(* Logix 5000 AddOnInstructionDefinition export Banner_Q90RKU_Param_v4; software revision 33.00; part 2 of 2 *)
(* tags used below, declared in another part *)
   Q90RKU : Banner_Q90RKU_v4;
   Port_Data : Banner_IOL_Port_v4;
   Port : DINT;
   Local_Control : DINT;
   Command_Being_Processed : BOOL;
   Update_Archive : BOOL;
   Index_Write_Inprocess : DINT;
   Index_Write_Control : DINT;
   Inprocess_Index : DINT;
(* Banner_Q90RKU_Param_v4, continued *)

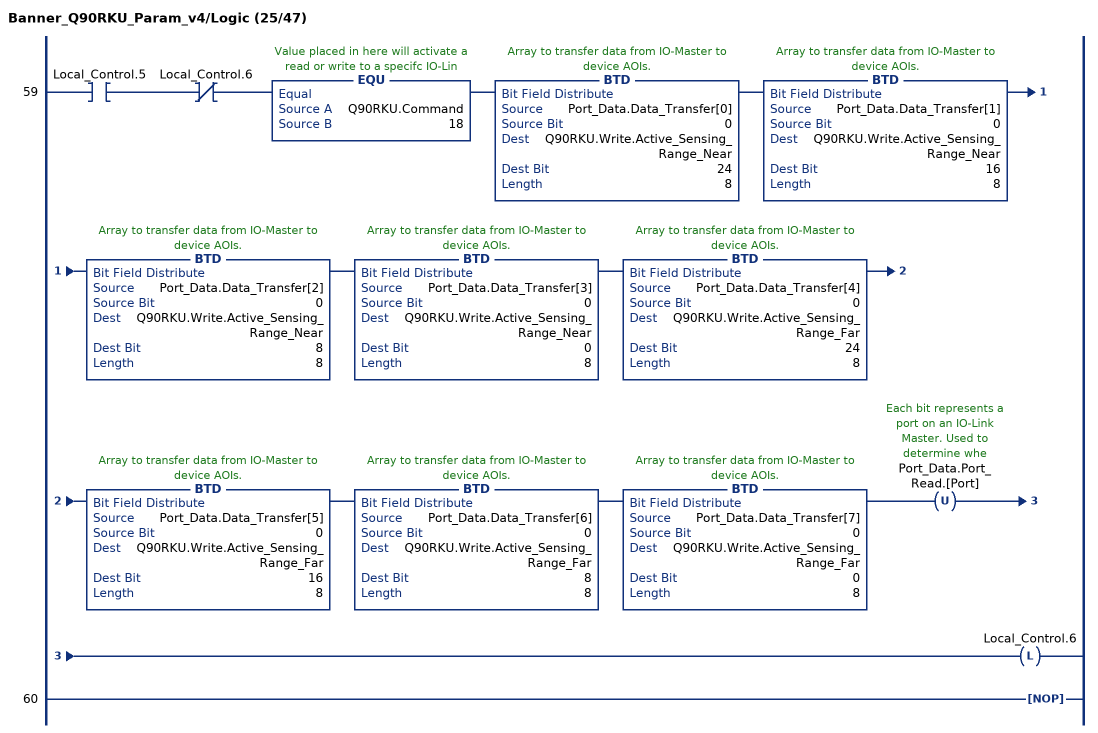
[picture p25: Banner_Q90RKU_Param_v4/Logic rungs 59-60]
   59: XIC(Local_Control.5)XIO(Local_Control.6)EQU(Q90RKU.Command,18)BTD(Port_Data.Data_Transfer[0],0,Q90RKU.Write.Active_Sensing_Range_Near,24,8)BTD(Port_Data.Data_Transfer[1],0,Q90RKU.Write.Active_Sensing_Range_Near,16,8)BTD(Port_Data.Data_Transfer[2],0,Q90RKU.Write.Active_Sensing_Range_Near,8,8)BTD(Port_Data.Data_Transfer[3],0,Q90RKU.Write.Active_Sensing_Range_Near,0,8)BTD(Port_Data.Data_Transfer[4],0,Q90RKU.Write.Active_Sensing_Range_Far,24,8)BTD(Port_Data.Data_Transfer[5],0,Q90RKU.Write.Active_Sensing_Range_Far,16,8)BTD(Port_Data.Data_Transfer[6],0,Q90RKU.Write.Active_Sensing_Range_Far,8,8)BTD(Port_Data.Data_Transfer[7],0,Q90RKU.Write.Active_Sensing_Range_Far,0,8)OTU(Port_Data.Port_Read.[Port])OTL(Local_Control.6);
   60: NOP();
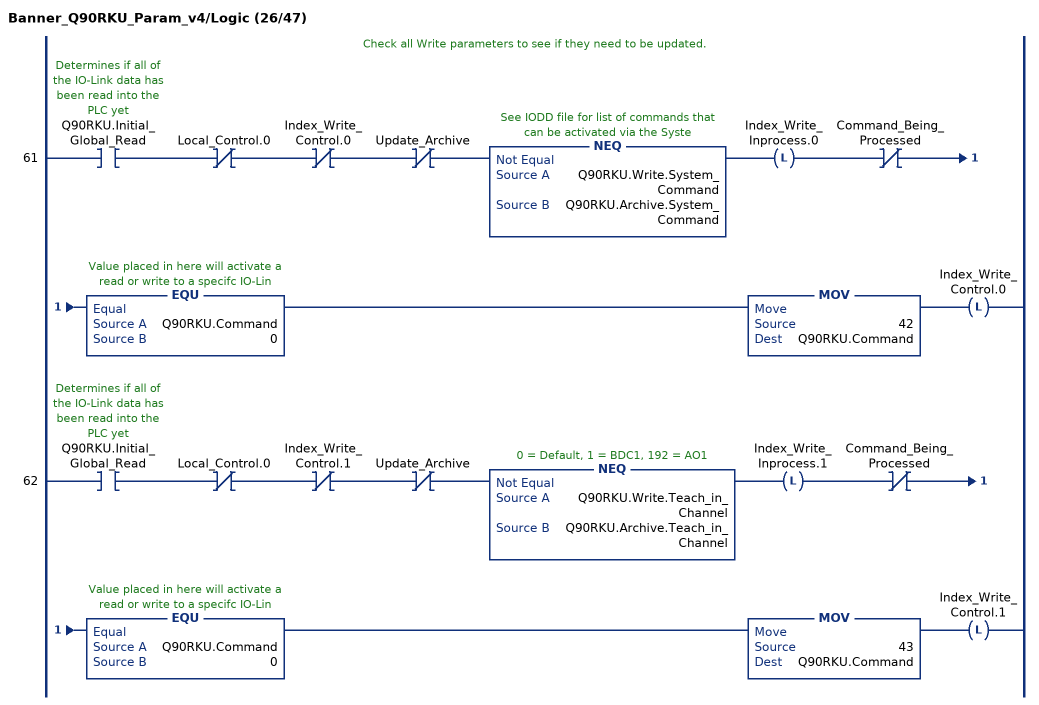
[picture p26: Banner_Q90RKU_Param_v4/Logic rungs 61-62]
   // Check all Write parameters to see if they need to be updated.
   61: XIC(Q90RKU.Initial_Global_Read)XIO(Local_Control.0)XIO(Index_Write_Control.0)XIO(Update_Archive)NEQ(Q90RKU.Write.System_Command,Q90RKU.Archive.System_Command)OTL(Index_Write_Inprocess.0)XIO(Command_Being_Processed)EQU(Q90RKU.Command,0)MOV(42,Q90RKU.Command)OTL(Index_Write_Control.0);
   62: XIC(Q90RKU.Initial_Global_Read)XIO(Local_Control.0)XIO(Index_Write_Control.1)XIO(Update_Archive)NEQ(Q90RKU.Write.Teach_in_Channel,Q90RKU.Archive.Teach_in_Channel)OTL(Index_Write_Inprocess.1)XIO(Command_Being_Processed)EQU(Q90RKU.Command,0)MOV(43,Q90RKU.Command)OTL(Index_Write_Control.1);
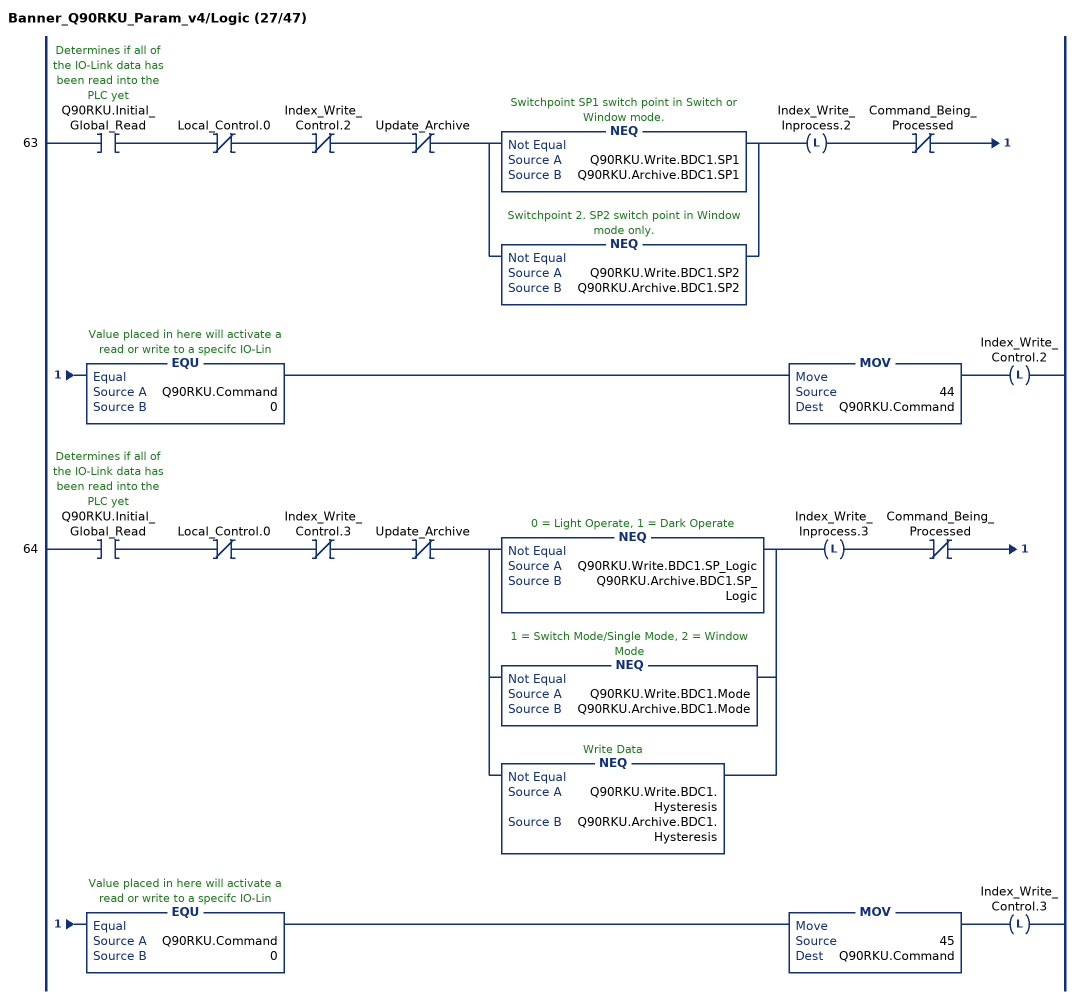
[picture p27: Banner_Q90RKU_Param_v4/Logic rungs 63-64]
   63: XIC(Q90RKU.Initial_Global_Read)XIO(Local_Control.0)XIO(Index_Write_Control.2)XIO(Update_Archive)[NEQ(Q90RKU.Write.BDC1.SP1,Q90RKU.Archive.BDC1.SP1) ,NEQ(Q90RKU.Write.BDC1.SP2,Q90RKU.Archive.BDC1.SP2) ]OTL(Index_Write_Inprocess.2)XIO(Command_Being_Processed)EQU(Q90RKU.Command,0)MOV(44,Q90RKU.Command)OTL(Index_Write_Control.2);
   64: XIC(Q90RKU.Initial_Global_Read)XIO(Local_Control.0)XIO(Index_Write_Control.3)XIO(Update_Archive)[NEQ(Q90RKU.Write.BDC1.SP_Logic,Q90RKU.Archive.BDC1.SP_Logic) ,NEQ(Q90RKU.Write.BDC1.Mode,Q90RKU.Archive.BDC1.Mode) ,NEQ(Q90RKU.Write.BDC1.Hysteresis,Q90RKU.Archive.BDC1.Hysteresis) ]OTL(Index_Write_Inprocess.3)XIO(Command_Being_Processed)EQU(Q90RKU.Command,0)MOV(45,Q90RKU.Command)OTL(Index_Write_Control.3);
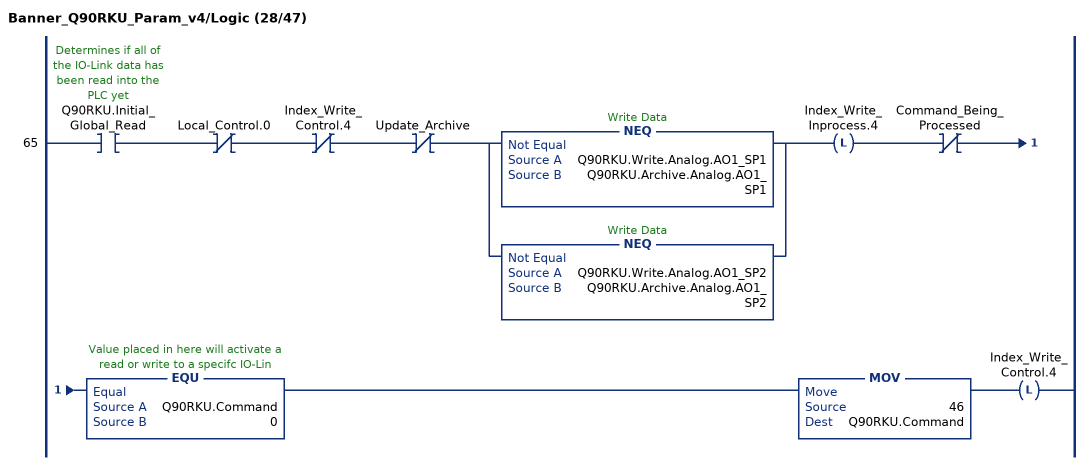
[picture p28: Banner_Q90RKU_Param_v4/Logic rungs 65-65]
   65: XIC(Q90RKU.Initial_Global_Read)XIO(Local_Control.0)XIO(Index_Write_Control.4)XIO(Update_Archive)[NEQ(Q90RKU.Write.Analog.AO1_SP1,Q90RKU.Archive.Analog.AO1_SP1) ,NEQ(Q90RKU.Write.Analog.AO1_SP2,Q90RKU.Archive.Analog.AO1_SP2) ]OTL(Index_Write_Inprocess.4)XIO(Command_Being_Processed)EQU(Q90RKU.Command,0)MOV(46,Q90RKU.Command)OTL(Index_Write_Control.4);
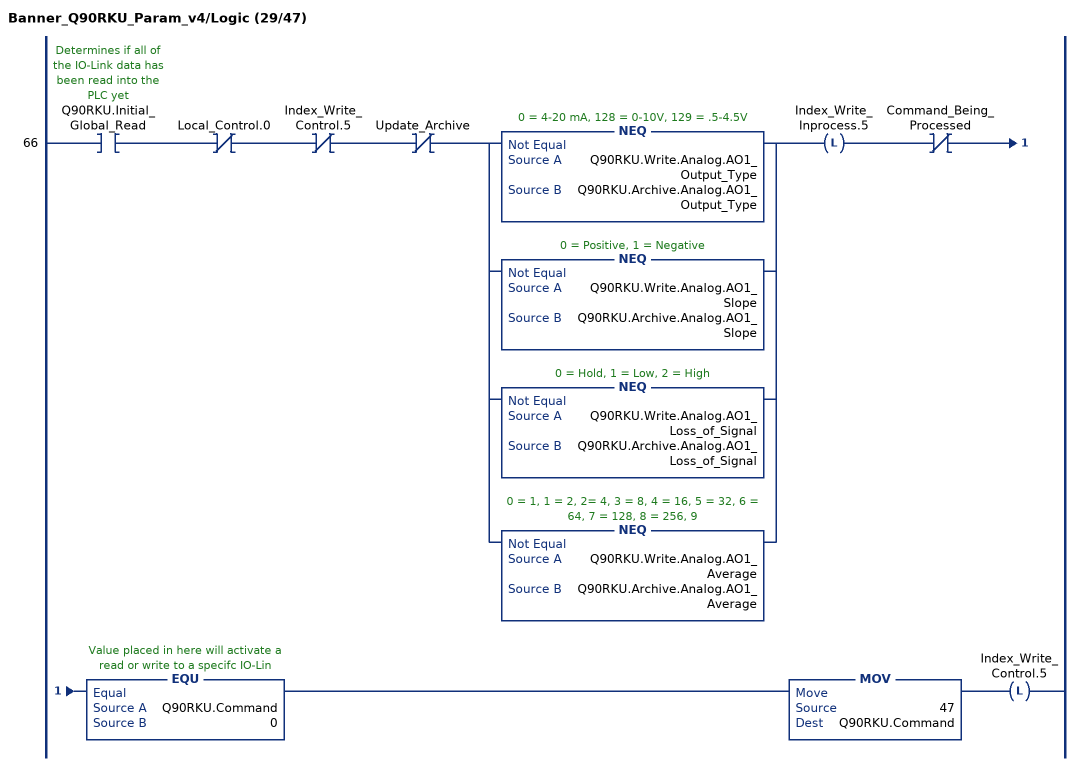
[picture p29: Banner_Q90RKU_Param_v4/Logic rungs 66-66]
   66: XIC(Q90RKU.Initial_Global_Read)XIO(Local_Control.0)XIO(Index_Write_Control.5)XIO(Update_Archive)[NEQ(Q90RKU.Write.Analog.AO1_Output_Type,Q90RKU.Archive.Analog.AO1_Output_Type) ,NEQ(Q90RKU.Write.Analog.AO1_Slope,Q90RKU.Archive.Analog.AO1_Slope) ,NEQ(Q90RKU.Write.Analog.AO1_Loss_of_Signal,Q90RKU.Archive.Analog.AO1_Loss_of_Signal) ,NEQ(Q90RKU.Write.Analog.AO1_Average,Q90RKU.Archive.Analog.AO1_Average) ]OTL(Index_Write_Inprocess.5)XIO(Command_Being_Processed)EQU(Q90RKU.Command,0)MOV(47,Q90RKU.Command)OTL(Index_Write_Control.5);
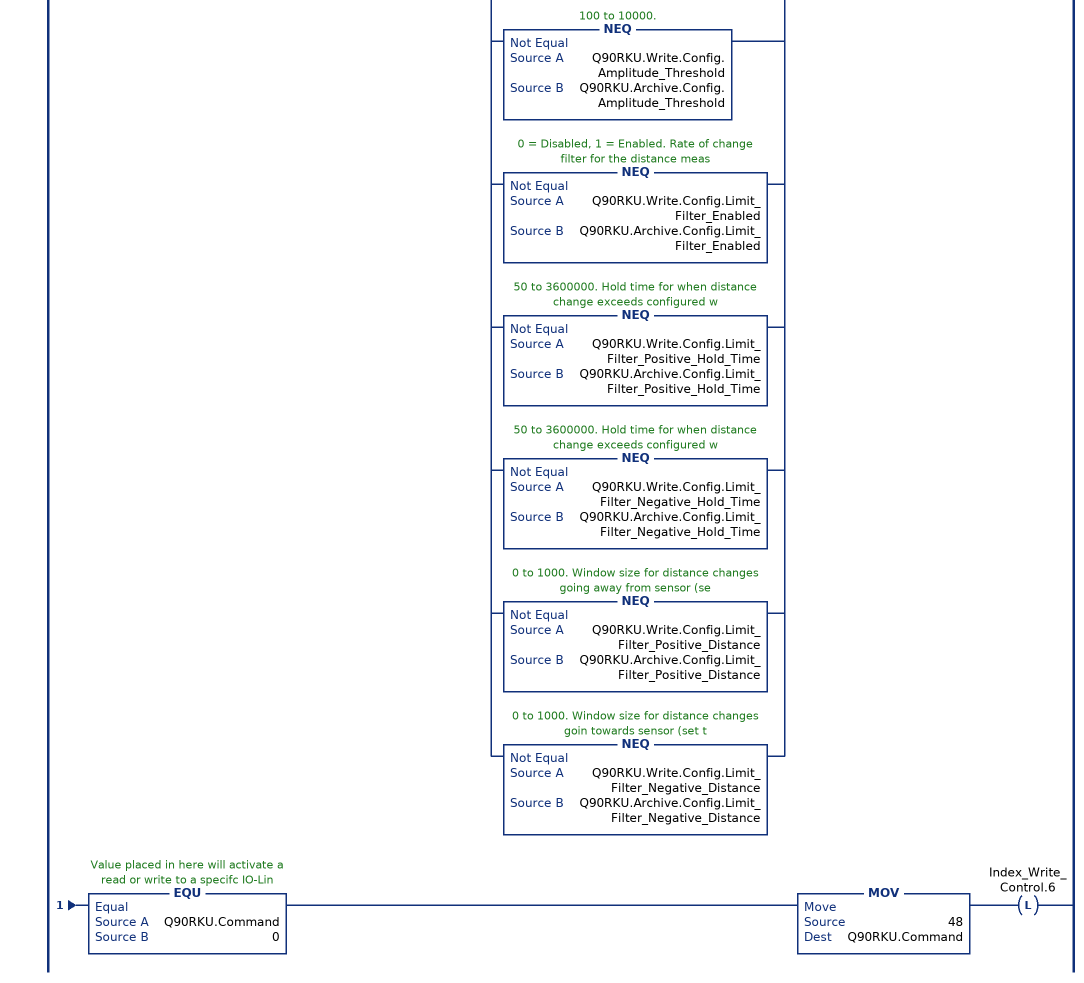
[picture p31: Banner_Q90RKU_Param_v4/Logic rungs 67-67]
   67: XIC(Q90RKU.Initial_Global_Read)XIO(Local_Control.0)XIO(Index_Write_Control.6)XIO(Update_Archive)[NEQ(Q90RKU.Write.Config.Response_Speed,Q90RKU.Archive.Config.Response_Speed) ,NEQ(Q90RKU.Write.Config.Peak_Select_Mode,Q90RKU.Archive.Config.Peak_Select_Mode) ,NEQ(Q90RKU.Write.Config.Output_Polarity,Q90RKU.Archive.Config.Output_Polarity) ,NEQ(Q90RKU.Write.Config.Process_Data_Filter_Time,Q90RKU.Archive.Config.Process_Data_Filter_Time) ,NEQ(Q90RKU.Write.Config.Process_Data_Layout,Q90RKU.Archive.Config.Process_Data_Layout) ,NEQ(Q90RKU.Write.Config.Remote_Input_Mode,Q90RKU.Archive.Config.Remote_Input_Mode) ,NEQ(Q90RKU.Write.Config.LEDs_Disabled,Q90RKU.Archive.Config.LEDs_Disabled) ,NEQ(Q90RKU.Write.Config.Amplitude_Threshold,Q90RKU.Archive.Config.Amplitude_Threshold) ,NEQ(Q90RKU.Write.Config.Limit_Filter_Enabled,Q90RKU.Archive.Config.Limit_Filter_Enabled) ,NEQ(Q90RKU.Write.Config.Limit_Filter_Positive_Hold_Time,Q90RKU.Archive.Config.Limit_Filter_Positive_Hold_Time) ,NEQ(Q90RKU.Write.Config.Limit_Filter_Negative_Hold_Time,Q90RKU.Archive.Config.Limit_Filter_Negative_Hold_Time) ,NEQ(Q90RKU.Write.Config.Limit_Filter_Positive_Distance,Q90RKU.Archive.Config.Limit_Filter_Positive_Distance) ,NEQ(Q90RKU.Write.Config.Limit_Filter_Negative_Distance,Q90RKU.Archive.Config.Limit_Filter_Negative_Distance) ]OTL(Index_Write_Inprocess.6)XIO(Command_Being_Processed)EQU(Q90RKU.Command,0)MOV(48,Q90RKU.Command)OTL(Index_Write_Control.6);
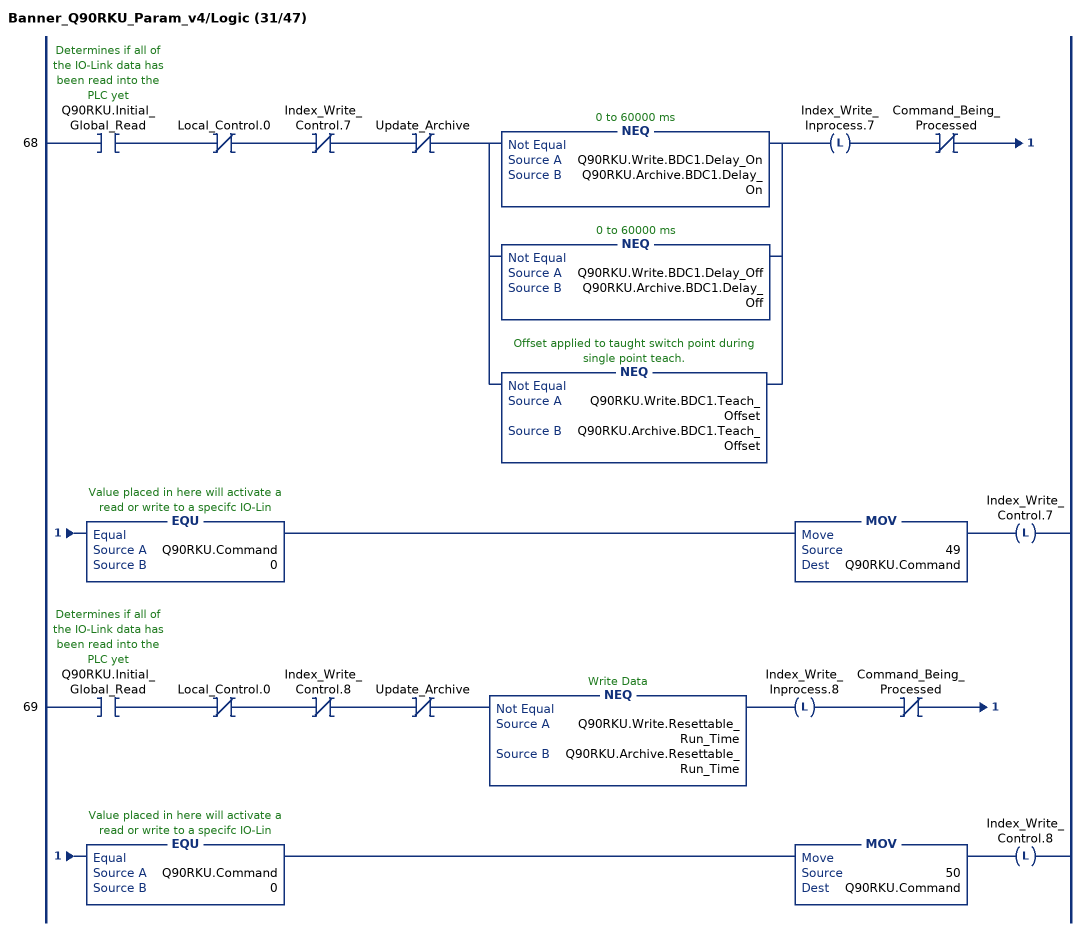
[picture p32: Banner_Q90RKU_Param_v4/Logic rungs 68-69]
   68: XIC(Q90RKU.Initial_Global_Read)XIO(Local_Control.0)XIO(Index_Write_Control.7)XIO(Update_Archive)[NEQ(Q90RKU.Write.BDC1.Delay_On,Q90RKU.Archive.BDC1.Delay_On) ,NEQ(Q90RKU.Write.BDC1.Delay_Off,Q90RKU.Archive.BDC1.Delay_Off) ,NEQ(Q90RKU.Write.BDC1.Teach_Offset,Q90RKU.Archive.BDC1.Teach_Offset) ]OTL(Index_Write_Inprocess.7)XIO(Command_Being_Processed)EQU(Q90RKU.Command,0)MOV(49,Q90RKU.Command)OTL(Index_Write_Control.7);
   69: XIC(Q90RKU.Initial_Global_Read)XIO(Local_Control.0)XIO(Index_Write_Control.8)XIO(Update_Archive)NEQ(Q90RKU.Write.Resettable_Run_Time,Q90RKU.Archive.Resettable_Run_Time)OTL(Index_Write_Inprocess.8)XIO(Command_Being_Processed)EQU(Q90RKU.Command,0)MOV(50,Q90RKU.Command)OTL(Index_Write_Control.8);
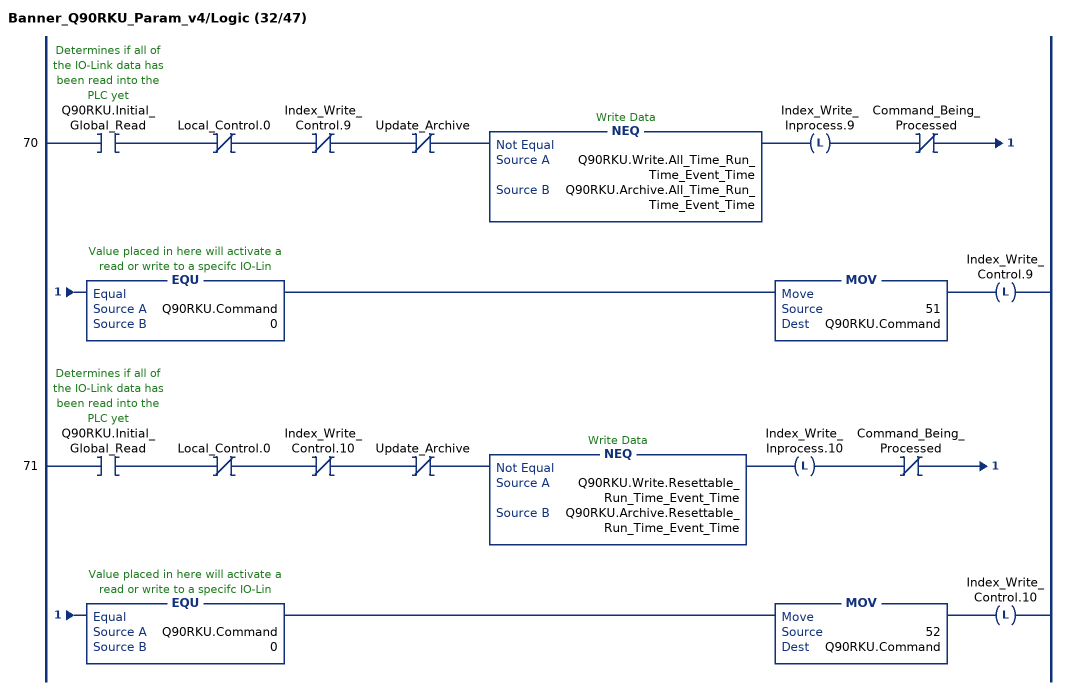
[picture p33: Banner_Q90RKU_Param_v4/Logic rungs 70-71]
   70: XIC(Q90RKU.Initial_Global_Read)XIO(Local_Control.0)XIO(Index_Write_Control.9)XIO(Update_Archive)NEQ(Q90RKU.Write.All_Time_Run_Time_Event_Time,Q90RKU.Archive.All_Time_Run_Time_Event_Time)OTL(Index_Write_Inprocess.9)XIO(Command_Being_Processed)EQU(Q90RKU.Command,0)MOV(51,Q90RKU.Command)OTL(Index_Write_Control.9);
   71: XIC(Q90RKU.Initial_Global_Read)XIO(Local_Control.0)XIO(Index_Write_Control.10)XIO(Update_Archive)NEQ(Q90RKU.Write.Resettable_Run_Time_Event_Time,Q90RKU.Archive.Resettable_Run_Time_Event_Time)OTL(Index_Write_Inprocess.10)XIO(Command_Being_Processed)EQU(Q90RKU.Command,0)MOV(52,Q90RKU.Command)OTL(Index_Write_Control.10);
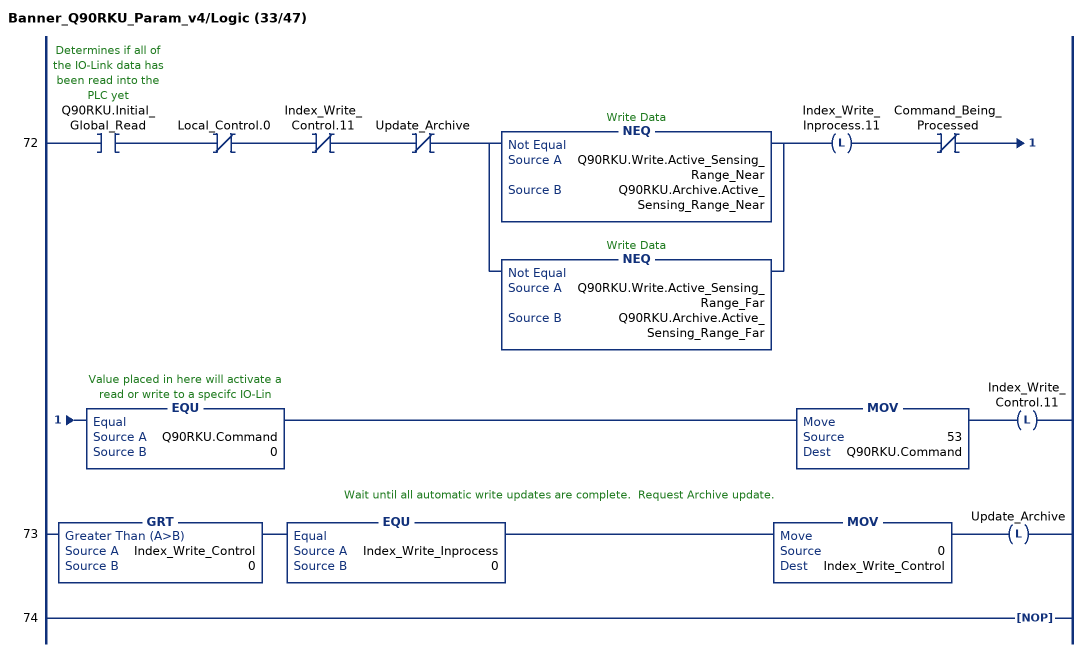
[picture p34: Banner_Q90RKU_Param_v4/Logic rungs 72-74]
   72: XIC(Q90RKU.Initial_Global_Read)XIO(Local_Control.0)XIO(Index_Write_Control.11)XIO(Update_Archive)[NEQ(Q90RKU.Write.Active_Sensing_Range_Near,Q90RKU.Archive.Active_Sensing_Range_Near) ,NEQ(Q90RKU.Write.Active_Sensing_Range_Far,Q90RKU.Archive.Active_Sensing_Range_Far) ]OTL(Index_Write_Inprocess.11)XIO(Command_Being_Processed)EQU(Q90RKU.Command,0)MOV(53,Q90RKU.Command)OTL(Index_Write_Control.11);
   // Wait until all automatic write updates are complete.  Request Archive update.
   73: GRT(Index_Write_Control,0)EQU(Index_Write_Inprocess,0)MOV(0,Index_Write_Control)OTL(Update_Archive);
   74: NOP();
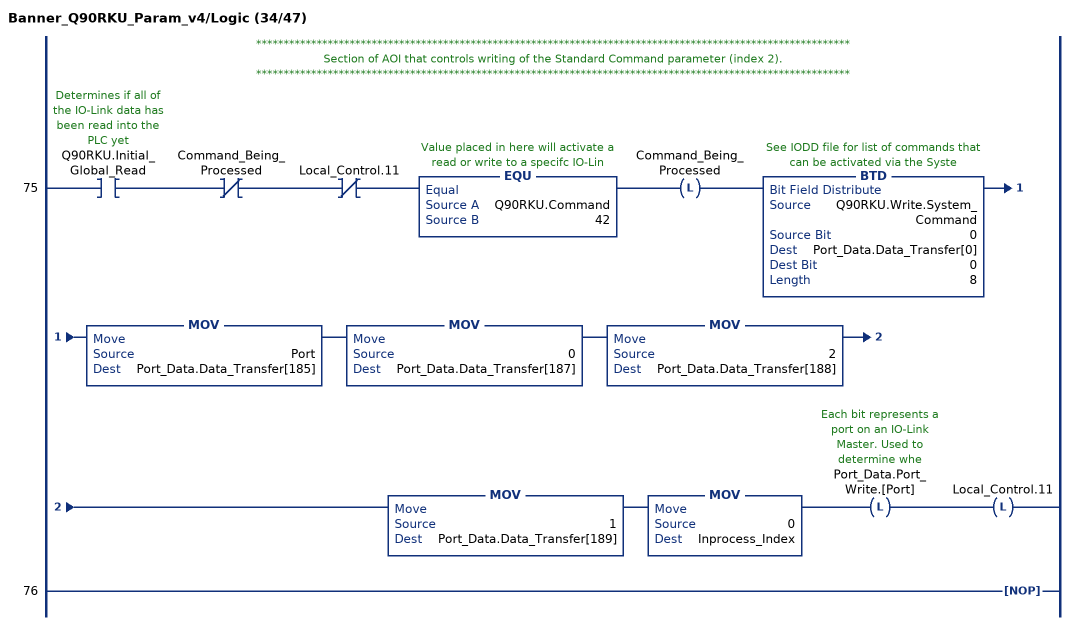
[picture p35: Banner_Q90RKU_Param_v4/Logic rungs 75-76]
   // ************************************************************************************************************
   // Section of AOI that controls writing of the Standard Command parameter (index 2).
   // ************************************************************************************************************
   75: XIC(Q90RKU.Initial_Global_Read)XIO(Command_Being_Processed)XIO(Local_Control.11)EQU(Q90RKU.Command,42)OTL(Command_Being_Processed)BTD(Q90RKU.Write.System_Command,0,Port_Data.Data_Transfer[0],0,8)MOV(Port,Port_Data.Data_Transfer[185])MOV(0,Port_Data.Data_Transfer[187])MOV(2,Port_Data.Data_Transfer[188])MOV(1,Port_Data.Data_Transfer[189])MOV(0,Inprocess_Index)OTL(Port_Data.Port_Write.[Port])OTL(Local_Control.11);
   76: NOP();
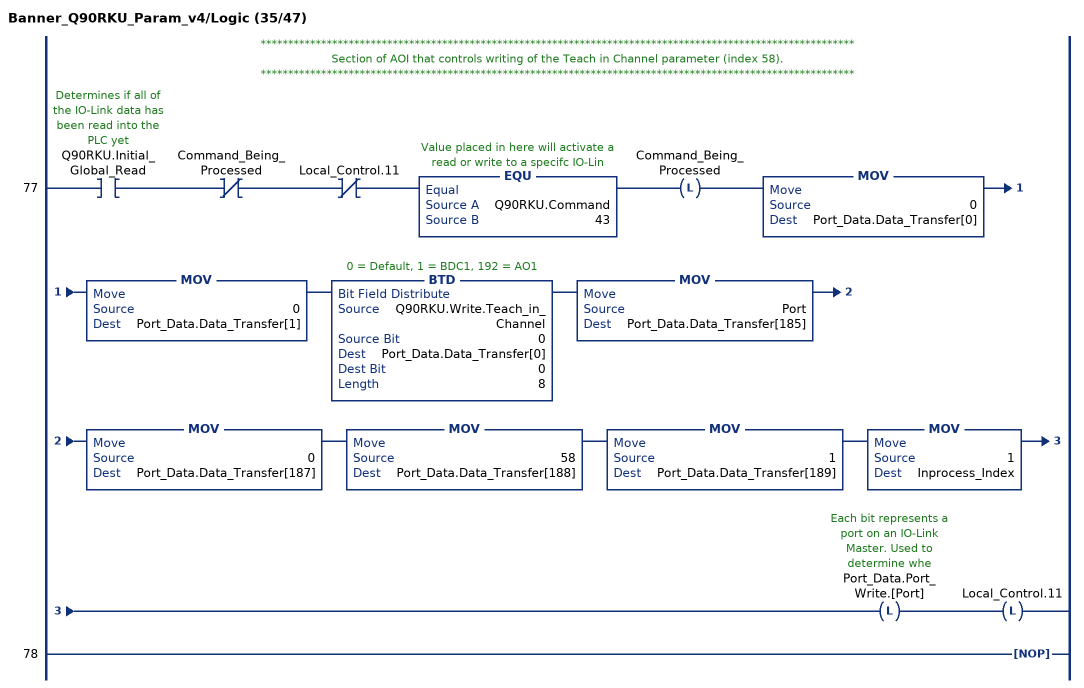
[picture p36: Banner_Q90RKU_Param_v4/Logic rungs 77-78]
   // ************************************************************************************************************
   // Section of AOI that controls writing of the Teach in Channel parameter (index 58).
   // ************************************************************************************************************
   77: XIC(Q90RKU.Initial_Global_Read)XIO(Command_Being_Processed)XIO(Local_Control.11)EQU(Q90RKU.Command,43)OTL(Command_Being_Processed)MOV(0,Port_Data.Data_Transfer[0])MOV(0,Port_Data.Data_Transfer[1])BTD(Q90RKU.Write.Teach_in_Channel,0,Port_Data.Data_Transfer[0],0,8)MOV(Port,Port_Data.Data_Transfer[185])MOV(0,Port_Data.Data_Transfer[187])MOV(58,Port_Data.Data_Transfer[188])MOV(1,Port_Data.Data_Transfer[189])MOV(1,Inprocess_Index)OTL(Port_Data.Port_Write.[Port])OTL(Local_Control.11);
   78: NOP();
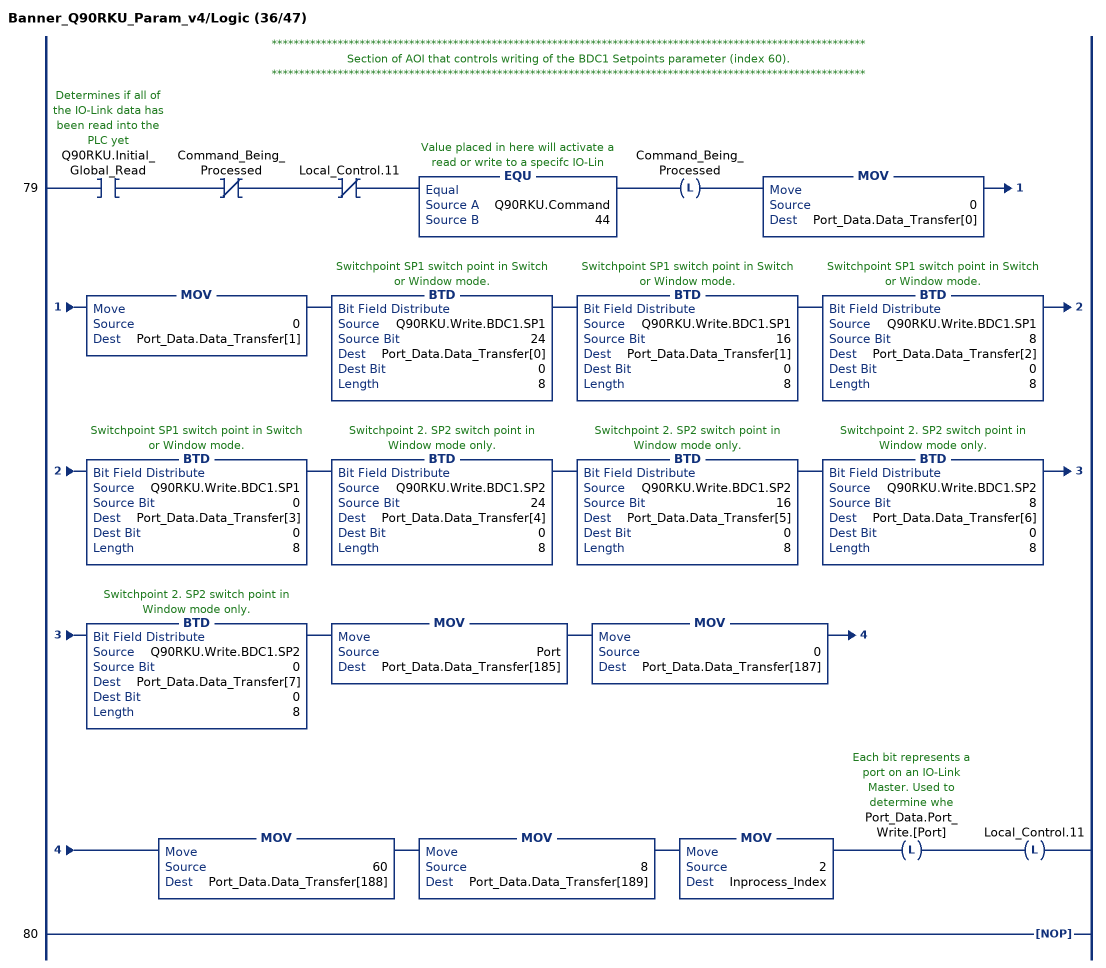
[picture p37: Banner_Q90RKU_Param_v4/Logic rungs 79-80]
   // ************************************************************************************************************
   // Section of AOI that controls writing of the BDC1 Setpoints parameter (index 60).
   // ************************************************************************************************************
   79: XIC(Q90RKU.Initial_Global_Read)XIO(Command_Being_Processed)XIO(Local_Control.11)EQU(Q90RKU.Command,44)OTL(Command_Being_Processed)MOV(0,Port_Data.Data_Transfer[0])MOV(0,Port_Data.Data_Transfer[1])BTD(Q90RKU.Write.BDC1.SP1,24,Port_Data.Data_Transfer[0],0,8)BTD(Q90RKU.Write.BDC1.SP1,16,Port_Data.Data_Transfer[1],0,8)BTD(Q90RKU.Write.BDC1.SP1,8,Port_Data.Data_Transfer[2],0,8)BTD(Q90RKU.Write.BDC1.SP1,0,Port_Data.Data_Transfer[3],0,8)BTD(Q90RKU.Write.BDC1.SP2,24,Port_Data.Data_Transfer[4],0,8)BTD(Q90RKU.Write.BDC1.SP2,16,Port_Data.Data_Transfer[5],0,8)BTD(Q90RKU.Write.BDC1.SP2,8,Port_Data.Data_Transfer[6],0,8)BTD(Q90RKU.Write.BDC1.SP2,0,Port_Data.Data_Transfer[7],0,8)MOV(Port,Port_Data.Data_Transfer[185])MOV(0,Port_Data.Data_Transfer[187])MOV(60,Port_Data.Data_Transfer[188])MOV(8,Port_Data.Data_Transfer[189])MOV(2,Inprocess_Index)OTL(Port_Data.Port_Write.[Port])OTL(Local_Control.11);
   80: NOP();
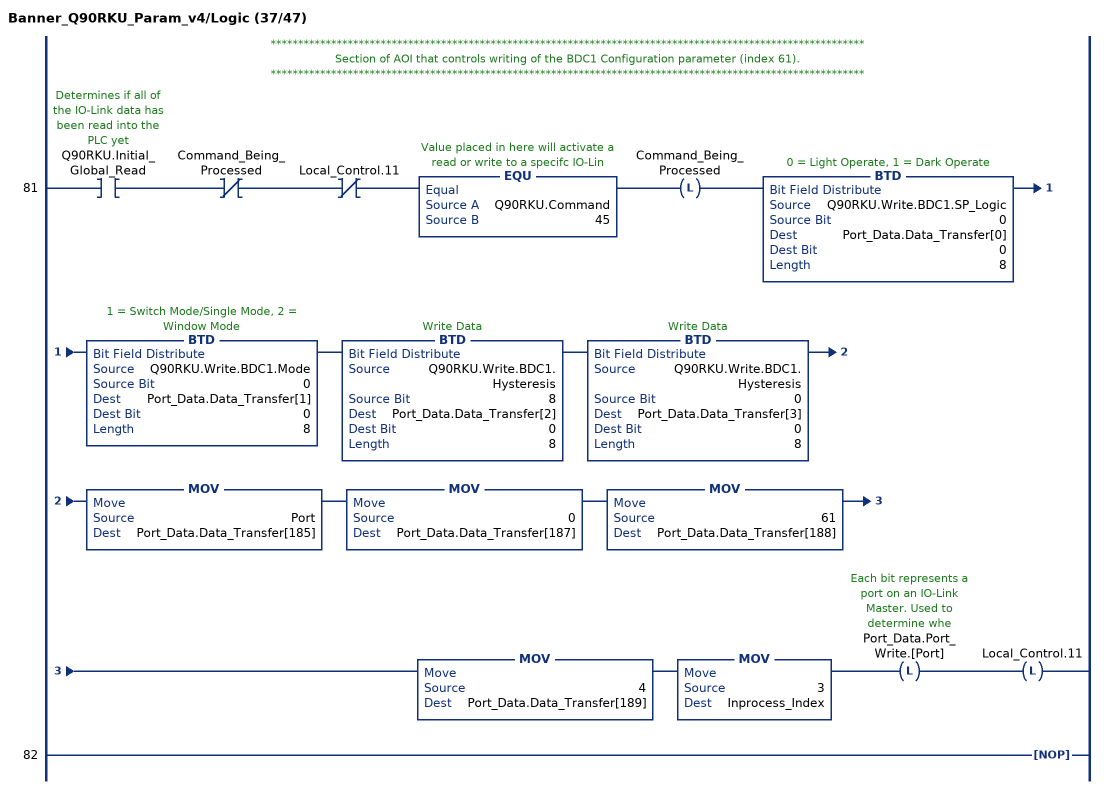
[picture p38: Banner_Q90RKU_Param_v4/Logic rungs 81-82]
   // ************************************************************************************************************
   // Section of AOI that controls writing of the BDC1 Configuration parameter (index 61).
   // ************************************************************************************************************
   81: XIC(Q90RKU.Initial_Global_Read)XIO(Command_Being_Processed)XIO(Local_Control.11)EQU(Q90RKU.Command,45)OTL(Command_Being_Processed)BTD(Q90RKU.Write.BDC1.SP_Logic,0,Port_Data.Data_Transfer[0],0,8)BTD(Q90RKU.Write.BDC1.Mode,0,Port_Data.Data_Transfer[1],0,8)BTD(Q90RKU.Write.BDC1.Hysteresis,8,Port_Data.Data_Transfer[2],0,8)BTD(Q90RKU.Write.BDC1.Hysteresis,0,Port_Data.Data_Transfer[3],0,8)MOV(Port,Port_Data.Data_Transfer[185])MOV(0,Port_Data.Data_Transfer[187])MOV(61,Port_Data.Data_Transfer[188])MOV(4,Port_Data.Data_Transfer[189])MOV(3,Inprocess_Index)OTL(Port_Data.Port_Write.[Port])OTL(Local_Control.11);
   82: NOP();
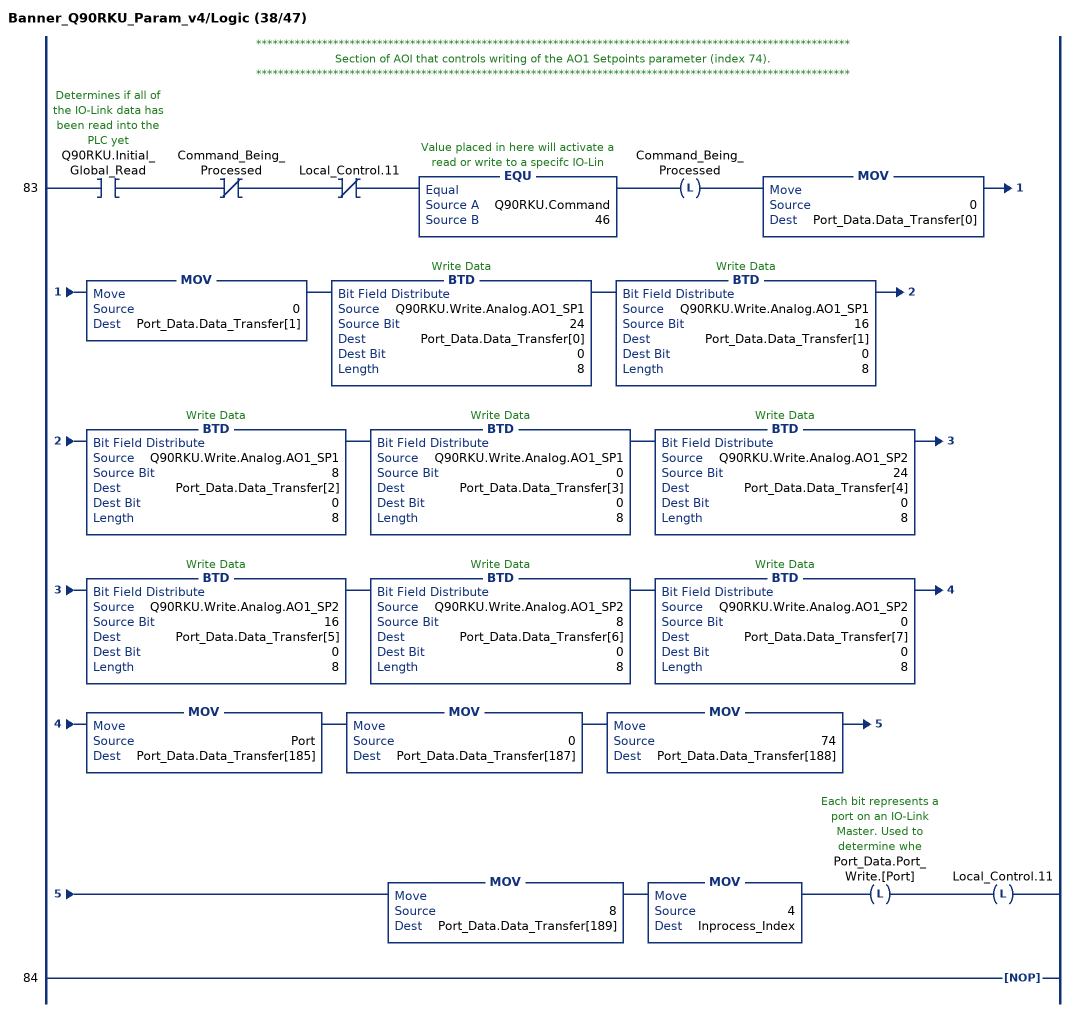
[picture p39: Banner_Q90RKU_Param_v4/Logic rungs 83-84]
   // ************************************************************************************************************
   // Section of AOI that controls writing of the AO1 Setpoints parameter (index 74).
   // ************************************************************************************************************
   83: XIC(Q90RKU.Initial_Global_Read)XIO(Command_Being_Processed)XIO(Local_Control.11)EQU(Q90RKU.Command,46)OTL(Command_Being_Processed)MOV(0,Port_Data.Data_Transfer[0])MOV(0,Port_Data.Data_Transfer[1])BTD(Q90RKU.Write.Analog.AO1_SP1,24,Port_Data.Data_Transfer[0],0,8)BTD(Q90RKU.Write.Analog.AO1_SP1,16,Port_Data.Data_Transfer[1],0,8)BTD(Q90RKU.Write.Analog.AO1_SP1,8,Port_Data.Data_Transfer[2],0,8)BTD(Q90RKU.Write.Analog.AO1_SP1,0,Port_Data.Data_Transfer[3],0,8)BTD(Q90RKU.Write.Analog.AO1_SP2,24,Port_Data.Data_Transfer[4],0,8)BTD(Q90RKU.Write.Analog.AO1_SP2,16,Port_Data.Data_Transfer[5],0,8)BTD(Q90RKU.Write.Analog.AO1_SP2,8,Port_Data.Data_Transfer[6],0,8)BTD(Q90RKU.Write.Analog.AO1_SP2,0,Port_Data.Data_Transfer[7],0,8)MOV(Port,Port_Data.Data_Transfer[185])MOV(0,Port_Data.Data_Transfer[187])MOV(74,Port_Data.Data_Transfer[188])MOV(8,Port_Data.Data_Transfer[189])MOV(4,Inprocess_Index)OTL(Port_Data.Port_Write.[Port])OTL(Local_Control.11);
   84: NOP();
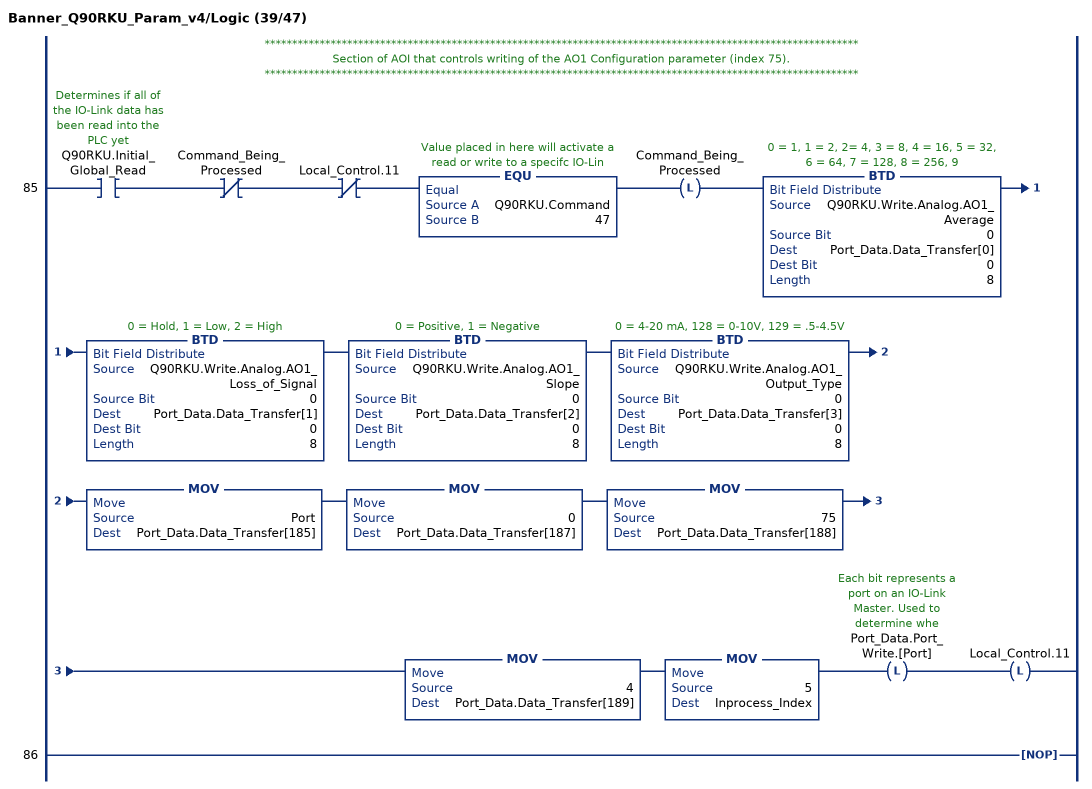
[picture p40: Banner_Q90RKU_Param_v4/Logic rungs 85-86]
   // ************************************************************************************************************
   // Section of AOI that controls writing of the AO1 Configuration parameter (index 75).
   // ************************************************************************************************************
   85: XIC(Q90RKU.Initial_Global_Read)XIO(Command_Being_Processed)XIO(Local_Control.11)EQU(Q90RKU.Command,47)OTL(Command_Being_Processed)BTD(Q90RKU.Write.Analog.AO1_Average,0,Port_Data.Data_Transfer[0],0,8)BTD(Q90RKU.Write.Analog.AO1_Loss_of_Signal,0,Port_Data.Data_Transfer[1],0,8)BTD(Q90RKU.Write.Analog.AO1_Slope,0,Port_Data.Data_Transfer[2],0,8)BTD(Q90RKU.Write.Analog.AO1_Output_Type,0,Port_Data.Data_Transfer[3],0,8)MOV(Port,Port_Data.Data_Transfer[185])MOV(0,Port_Data.Data_Transfer[187])MOV(75,Port_Data.Data_Transfer[188])MOV(4,Port_Data.Data_Transfer[189])MOV(5,Inprocess_Index)OTL(Port_Data.Port_Write.[Port])OTL(Local_Control.11);
   86: NOP();
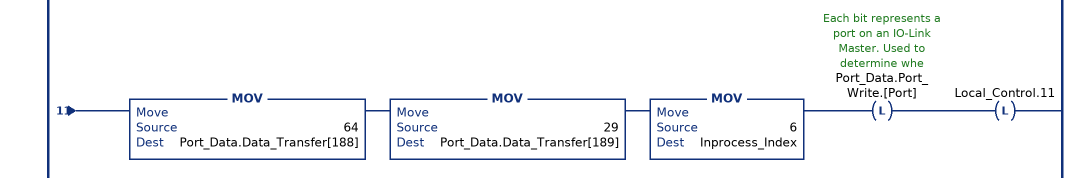
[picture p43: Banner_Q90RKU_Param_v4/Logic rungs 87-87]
   // ************************************************************************************************************
   // Section of AOI that controls writing of the Configuration parameter (index 64).
   // ************************************************************************************************************
   87: XIC(Q90RKU.Initial_Global_Read)XIO(Command_Being_Processed)XIO(Local_Control.11)EQU(Q90RKU.Command,48)OTL(Command_Being_Processed)BTD(Q90RKU.Write.Config.Response_Speed,0,Port_Data.Data_Transfer[0],0,8)BTD(Q90RKU.Write.Config.Peak_Select_Mode,0,Port_Data.Data_Transfer[1],0,8)BTD(Q90RKU.Write.Config.Output_Polarity,0,Port_Data.Data_Transfer[2],0,8)BTD(Q90RKU.Write.Config.Process_Data_Filter_Time,8,Port_Data.Data_Transfer[3],0,8)BTD(Q90RKU.Write.Config.Process_Data_Filter_Time,0,Port_Data.Data_Transfer[4],0,8)BTD(Q90RKU.Write.Config.Process_Data_Layout,0,Port_Data.Data_Transfer[5],0,8)BTD(Q90RKU.Write.Config.Remote_Input_Mode,0,Port_Data.Data_Transfer[6],0,8)BTD(Q90RKU.Write.Config.LEDs_Disabled,0,Port_Data.Data_Transfer[7],0,8)BTD(Q90RKU.Write.Config.Amplitude_Threshold,24,Port_Data.Data_Transfer[8],0,8)BTD(Q90RKU.Write.Config.Amplitude_Threshold,16,Port_Data.Data_Transfer[9],0,8)BTD(Q90RKU.Write.Config.Amplitude_Threshold,8,Port_Data.Data_Transfer[10],0,8)BTD(Q90RKU.Write.Config.Amplitude_Threshold,0,Port_Data.Data_Transfer[11],0,8)BTD(Q90RKU.Write.Config.Limit_Filter_Enabled,0,Port_Data.Data_Transfer[12],0,8)BTD(Q90RKU.Write.Config.Limit_Filter_Positive_Hold_Time,24,Port_Data.Data_Transfer[13],0,8)BTD(Q90RKU.Write.Config.Limit_Filter_Positive_Hold_Time,16,Port_Data.Data_Transfer[14],0,8)BTD(Q90RKU.Write.Config.Limit_Filter_Positive_Hold_Time,8,Port_Data.Data_Transfer[15],0,8)BTD(Q90RKU.Write.Config.Limit_Filter_Positive_Hold_Time,0,Port_Data.Data_Transfer[16],0,8)BTD(Q90RKU.Write.Config.Limit_Filter_Negative_Hold_Time,24,Port_Data.Data_Transfer[17],0,8)BTD(Q90RKU.Write.Config.Limit_Filter_Negative_Hold_Time,16,Port_Data.Data_Transfer[18],0,8)BTD(Q90RKU.Write.Config.Limit_Filter_Negative_Hold_Time,8,Port_Data.Data_Transfer[19],0,8)BTD(Q90RKU.Write.Config.Limit_Filter_Negative_Hold_Time,0,Port_Data.Data_Transfer[20],0,8)BTD(Q90RKU.Write.Config.Limit_Filter_Positive_Distance,24,Port_Data.Data_Transfer[21],0,8)BTD(Q90RKU.Write.Config.Limit_Filter_Positive_Distance,16,Port_Data.Data_Transfer[22],0,8)BTD(Q90RKU.Write.Config.Limit_Filter_Positive_Distance,8,Port_Data.Data_Transfer[23],0,8)BTD(Q90RKU.Write.Config.Limit_Filter_Positive_Distance,0,Port_Data.Data_Transfer[24],0,8)BTD(Q90RKU.Write.Config.Limit_Filter_Negative_Distance,24,Port_Data.Data_Transfer[25],0,8)BTD(Q90RKU.Write.Config.Limit_Filter_Negative_Distance,16,Port_Data.Data_Transfer[26],0,8)BTD(Q90RKU.Write.Config.Limit_Filter_Negative_Distance,8,Port_Data.Data_Transfer[27],0,8)BTD(Q90RKU.Write.Config.Limit_Filter_Negative_Distance,0,Port_Data.Data_Transfer[28],0,8)MOV(Port,Port_Data.Data_Transfer[185])MOV(0,Port_Data.Data_Transfer[187])MOV(64,Port_Data.Data_Transfer[188])MOV(29,Port_Data.Data_Transfer[189])MOV(6,Inprocess_Index)OTL(Port_Data.Port_Write.[Port])OTL(Local_Control.11);
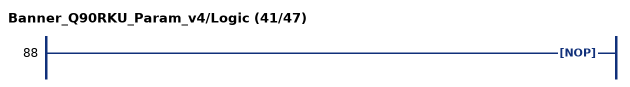
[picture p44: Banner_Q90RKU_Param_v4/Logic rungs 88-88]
   88: NOP();
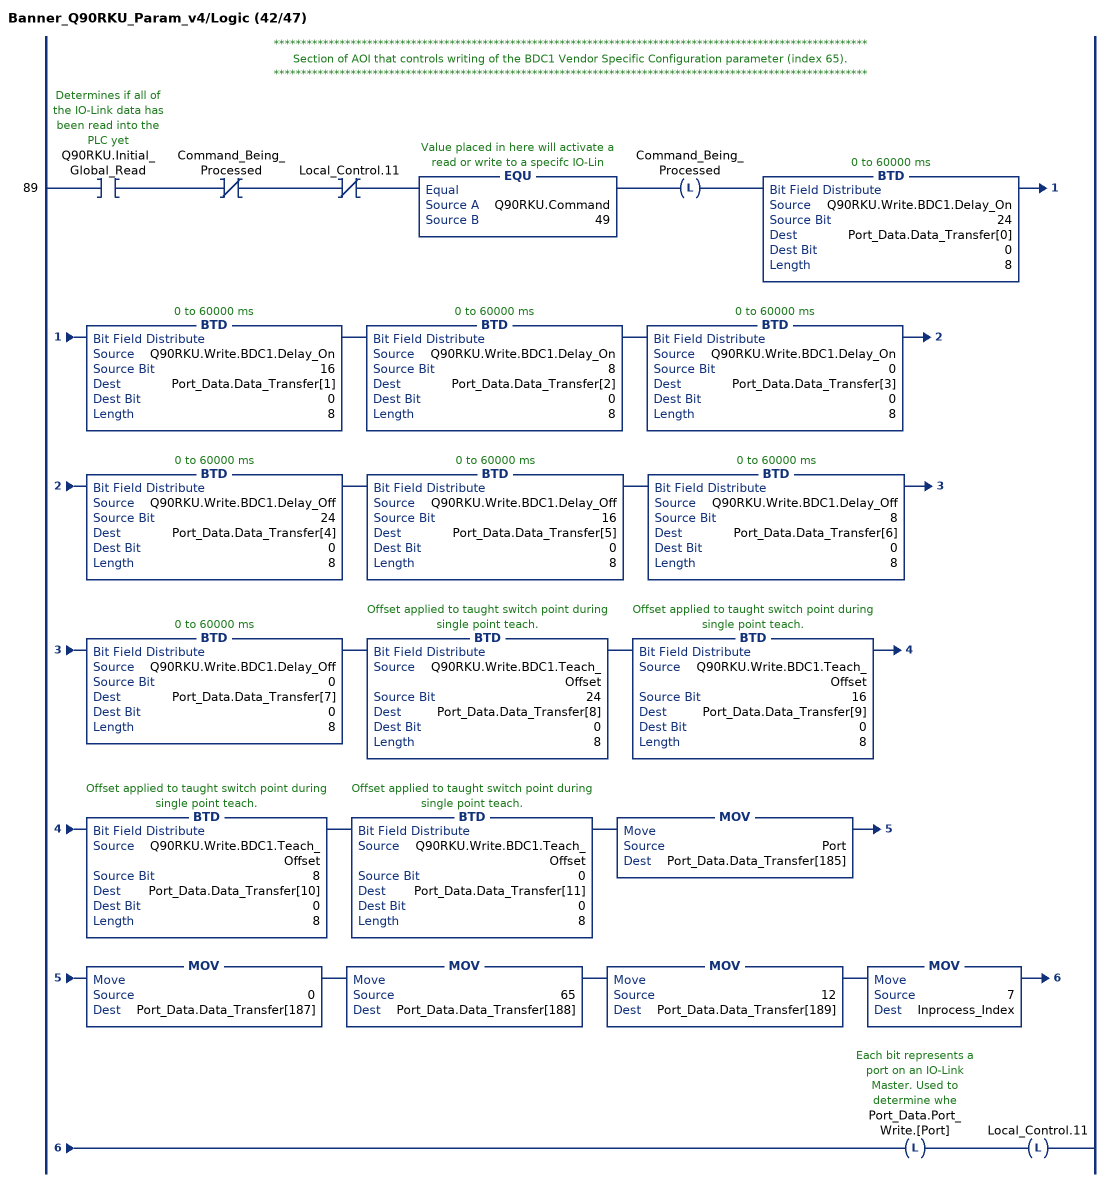
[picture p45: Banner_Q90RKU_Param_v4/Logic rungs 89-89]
   // ************************************************************************************************************
   // Section of AOI that controls writing of the BDC1 Vendor Specific Configuration parameter (index 65).
   // ************************************************************************************************************
   89: XIC(Q90RKU.Initial_Global_Read)XIO(Command_Being_Processed)XIO(Local_Control.11)EQU(Q90RKU.Command,49)OTL(Command_Being_Processed)BTD(Q90RKU.Write.BDC1.Delay_On,24,Port_Data.Data_Transfer[0],0,8)BTD(Q90RKU.Write.BDC1.Delay_On,16,Port_Data.Data_Transfer[1],0,8)BTD(Q90RKU.Write.BDC1.Delay_On,8,Port_Data.Data_Transfer[2],0,8)BTD(Q90RKU.Write.BDC1.Delay_On,0,Port_Data.Data_Transfer[3],0,8)BTD(Q90RKU.Write.BDC1.Delay_Off,24,Port_Data.Data_Transfer[4],0,8)BTD(Q90RKU.Write.BDC1.Delay_Off,16,Port_Data.Data_Transfer[5],0,8)BTD(Q90RKU.Write.BDC1.Delay_Off,8,Port_Data.Data_Transfer[6],0,8)BTD(Q90RKU.Write.BDC1.Delay_Off,0,Port_Data.Data_Transfer[7],0,8)BTD(Q90RKU.Write.BDC1.Teach_Offset,24,Port_Data.Data_Transfer[8],0,8)BTD(Q90RKU.Write.BDC1.Teach_Offset,16,Port_Data.Data_Transfer[9],0,8)BTD(Q90RKU.Write.BDC1.Teach_Offset,8,Port_Data.Data_Transfer[10],0,8)BTD(Q90RKU.Write.BDC1.Teach_Offset,0,Port_Data.Data_Transfer[11],0,8)MOV(Port,Port_Data.Data_Transfer[185])MOV(0,Port_Data.Data_Transfer[187])MOV(65,Port_Data.Data_Transfer[188])MOV(12,Port_Data.Data_Transfer[189])MOV(7,Inprocess_Index)OTL(Port_Data.Port_Write.[Port])OTL(Local_Control.11);
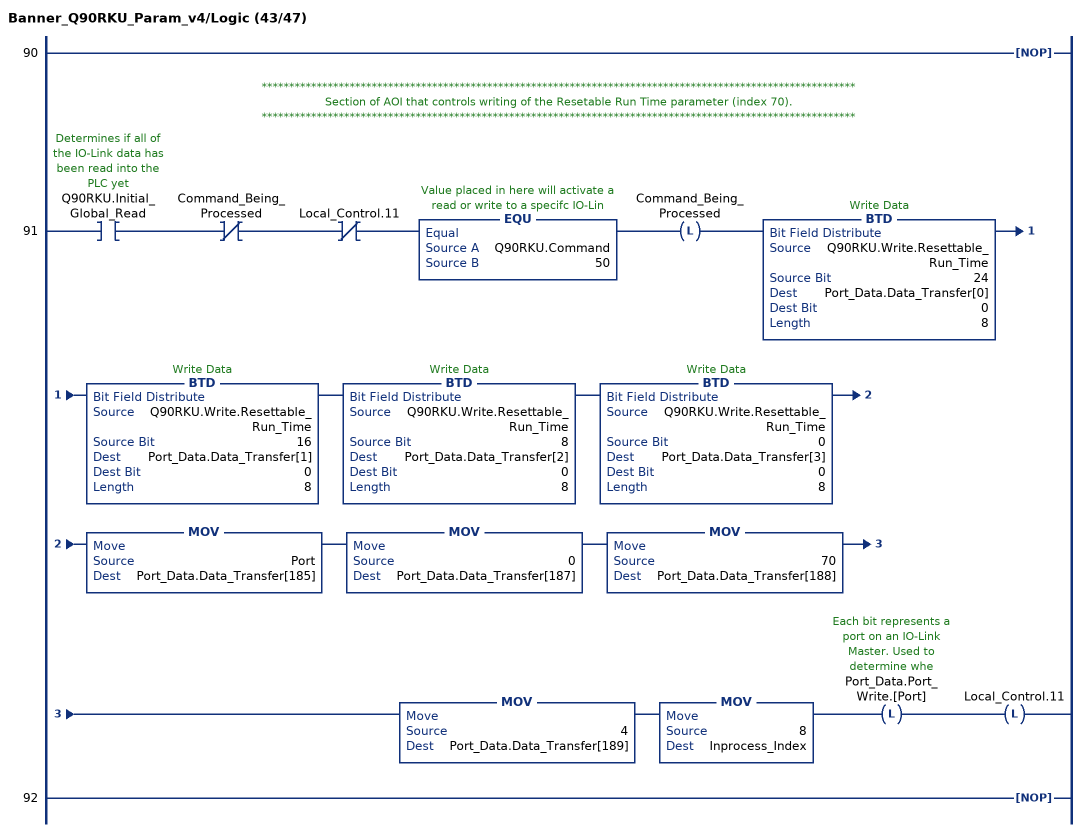
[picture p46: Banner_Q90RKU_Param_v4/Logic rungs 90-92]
   90: NOP();
   // ************************************************************************************************************
   // Section of AOI that controls writing of the Resetable Run Time parameter (index 70).
   // ************************************************************************************************************
   91: XIC(Q90RKU.Initial_Global_Read)XIO(Command_Being_Processed)XIO(Local_Control.11)EQU(Q90RKU.Command,50)OTL(Command_Being_Processed)BTD(Q90RKU.Write.Resettable_Run_Time,24,Port_Data.Data_Transfer[0],0,8)BTD(Q90RKU.Write.Resettable_Run_Time,16,Port_Data.Data_Transfer[1],0,8)BTD(Q90RKU.Write.Resettable_Run_Time,8,Port_Data.Data_Transfer[2],0,8)BTD(Q90RKU.Write.Resettable_Run_Time,0,Port_Data.Data_Transfer[3],0,8)MOV(Port,Port_Data.Data_Transfer[185])MOV(0,Port_Data.Data_Transfer[187])MOV(70,Port_Data.Data_Transfer[188])MOV(4,Port_Data.Data_Transfer[189])MOV(8,Inprocess_Index)OTL(Port_Data.Port_Write.[Port])OTL(Local_Control.11);
   92: NOP();
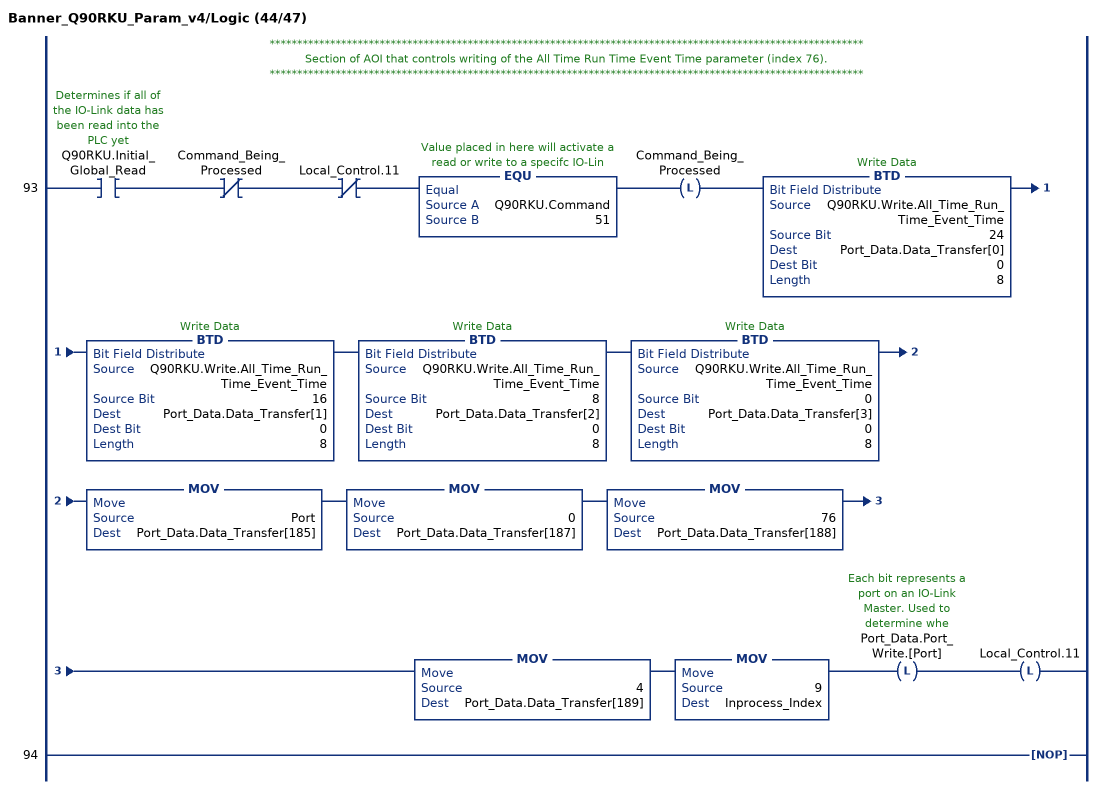
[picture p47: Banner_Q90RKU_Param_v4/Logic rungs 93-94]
   // ************************************************************************************************************
   // Section of AOI that controls writing of the All Time Run Time Event Time parameter (index 76).
   // ************************************************************************************************************
   93: XIC(Q90RKU.Initial_Global_Read)XIO(Command_Being_Processed)XIO(Local_Control.11)EQU(Q90RKU.Command,51)OTL(Command_Being_Processed)BTD(Q90RKU.Write.All_Time_Run_Time_Event_Time,24,Port_Data.Data_Transfer[0],0,8)BTD(Q90RKU.Write.All_Time_Run_Time_Event_Time,16,Port_Data.Data_Transfer[1],0,8)BTD(Q90RKU.Write.All_Time_Run_Time_Event_Time,8,Port_Data.Data_Transfer[2],0,8)BTD(Q90RKU.Write.All_Time_Run_Time_Event_Time,0,Port_Data.Data_Transfer[3],0,8)MOV(Port,Port_Data.Data_Transfer[185])MOV(0,Port_Data.Data_Transfer[187])MOV(76,Port_Data.Data_Transfer[188])MOV(4,Port_Data.Data_Transfer[189])MOV(9,Inprocess_Index)OTL(Port_Data.Port_Write.[Port])OTL(Local_Control.11);
   94: NOP();
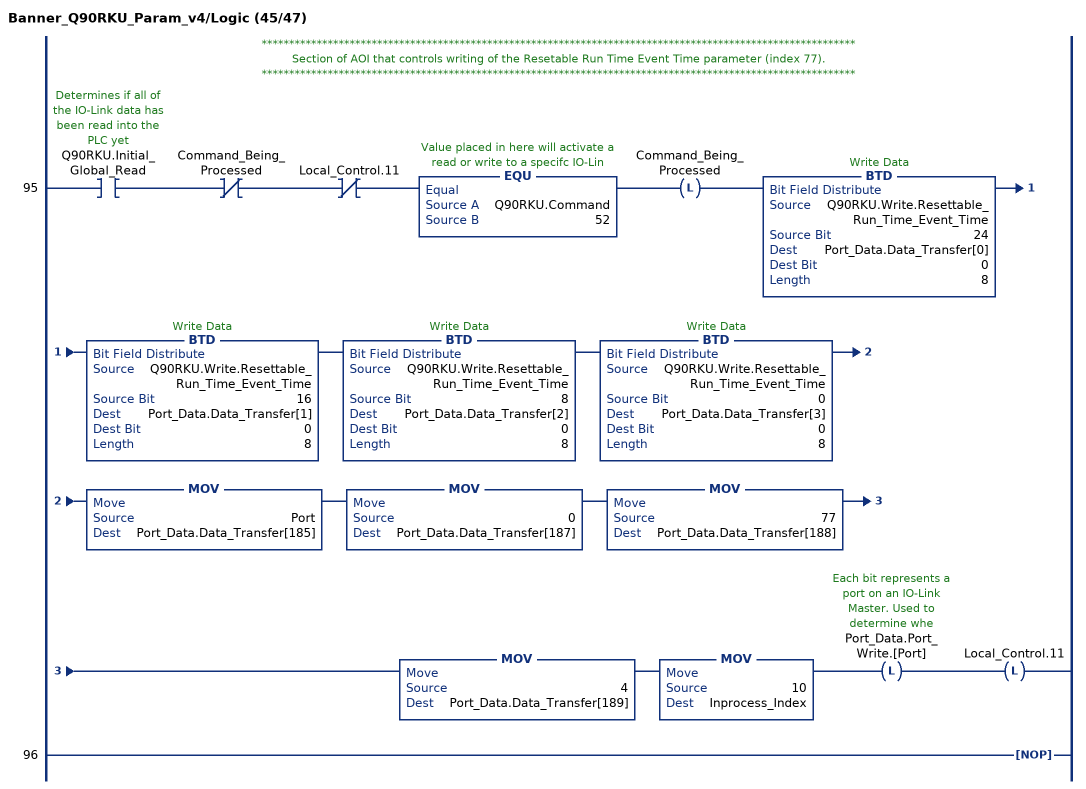
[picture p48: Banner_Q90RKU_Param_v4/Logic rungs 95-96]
   // ************************************************************************************************************
   // Section of AOI that controls writing of the Resetable Run Time Event Time parameter (index 77).
   // ************************************************************************************************************
   95: XIC(Q90RKU.Initial_Global_Read)XIO(Command_Being_Processed)XIO(Local_Control.11)EQU(Q90RKU.Command,52)OTL(Command_Being_Processed)BTD(Q90RKU.Write.Resettable_Run_Time_Event_Time,24,Port_Data.Data_Transfer[0],0,8)BTD(Q90RKU.Write.Resettable_Run_Time_Event_Time,16,Port_Data.Data_Transfer[1],0,8)BTD(Q90RKU.Write.Resettable_Run_Time_Event_Time,8,Port_Data.Data_Transfer[2],0,8)BTD(Q90RKU.Write.Resettable_Run_Time_Event_Time,0,Port_Data.Data_Transfer[3],0,8)MOV(Port,Port_Data.Data_Transfer[185])MOV(0,Port_Data.Data_Transfer[187])MOV(77,Port_Data.Data_Transfer[188])MOV(4,Port_Data.Data_Transfer[189])MOV(10,Inprocess_Index)OTL(Port_Data.Port_Write.[Port])OTL(Local_Control.11);
   96: NOP();
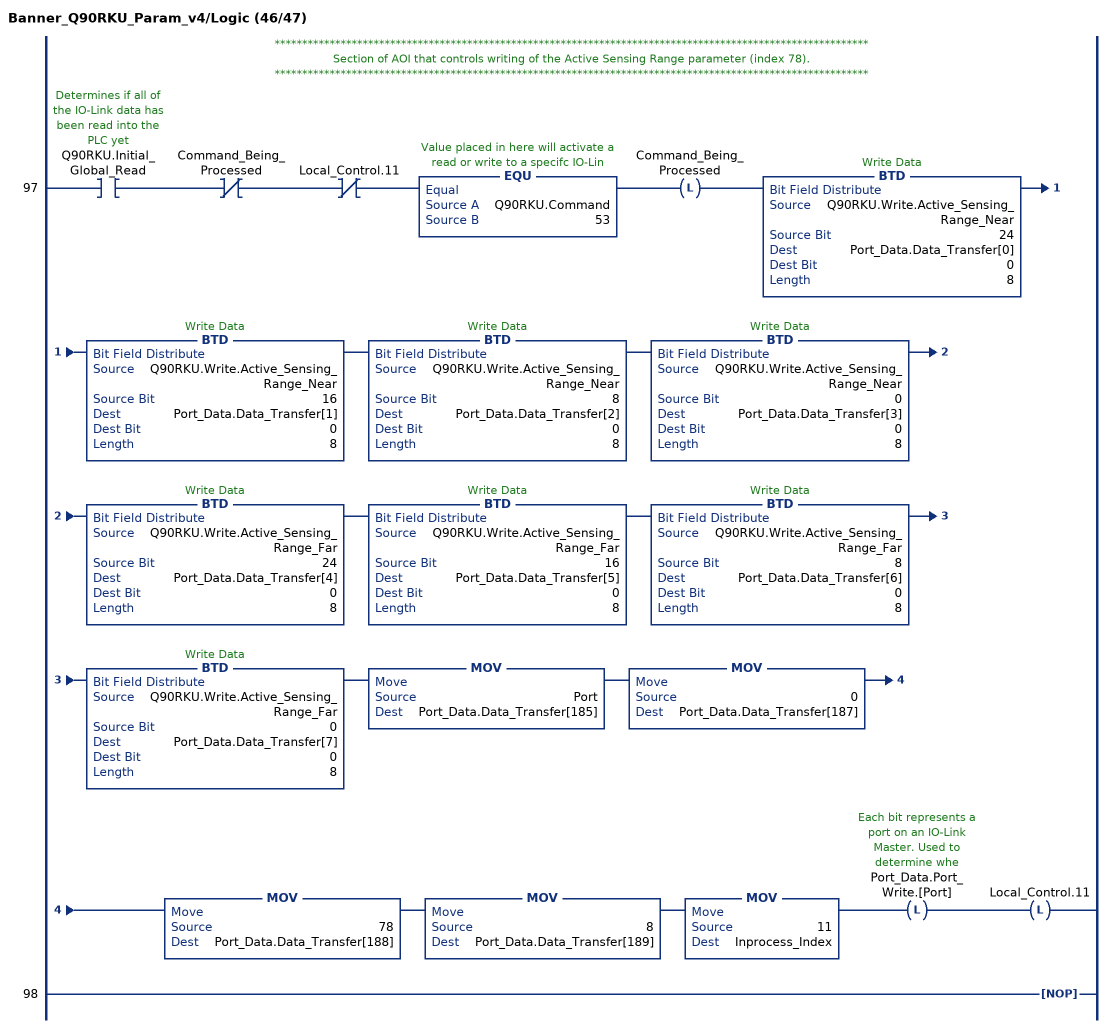
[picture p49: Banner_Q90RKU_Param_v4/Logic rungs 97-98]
   // ************************************************************************************************************
   // Section of AOI that controls writing of the Active Sensing Range parameter (index 78).
   // ************************************************************************************************************
   97: XIC(Q90RKU.Initial_Global_Read)XIO(Command_Being_Processed)XIO(Local_Control.11)EQU(Q90RKU.Command,53)OTL(Command_Being_Processed)BTD(Q90RKU.Write.Active_Sensing_Range_Near,24,Port_Data.Data_Transfer[0],0,8)BTD(Q90RKU.Write.Active_Sensing_Range_Near,16,Port_Data.Data_Transfer[1],0,8)BTD(Q90RKU.Write.Active_Sensing_Range_Near,8,Port_Data.Data_Transfer[2],0,8)BTD(Q90RKU.Write.Active_Sensing_Range_Near,0,Port_Data.Data_Transfer[3],0,8)BTD(Q90RKU.Write.Active_Sensing_Range_Far,24,Port_Data.Data_Transfer[4],0,8)BTD(Q90RKU.Write.Active_Sensing_Range_Far,16,Port_Data.Data_Transfer[5],0,8)BTD(Q90RKU.Write.Active_Sensing_Range_Far,8,Port_Data.Data_Transfer[6],0,8)BTD(Q90RKU.Write.Active_Sensing_Range_Far,0,Port_Data.Data_Transfer[7],0,8)MOV(Port,Port_Data.Data_Transfer[185])MOV(0,Port_Data.Data_Transfer[187])MOV(78,Port_Data.Data_Transfer[188])MOV(8,Port_Data.Data_Transfer[189])MOV(11,Inprocess_Index)OTL(Port_Data.Port_Write.[Port])OTL(Local_Control.11);
   98: NOP();
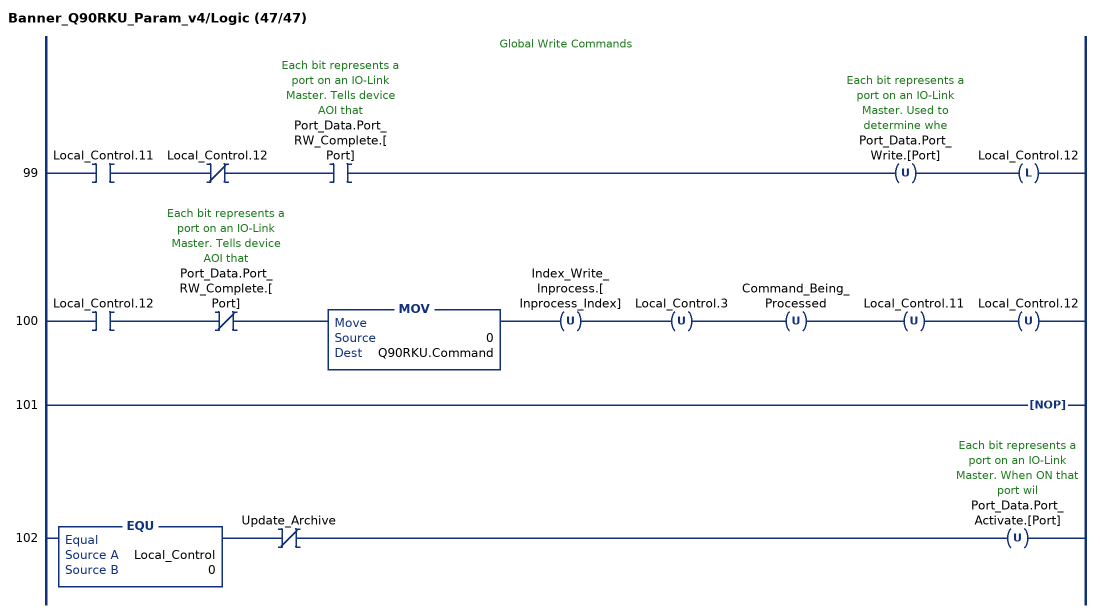
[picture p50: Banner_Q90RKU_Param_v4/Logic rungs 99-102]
   // Global Write Commands
   99: XIC(Local_Control.11)XIO(Local_Control.12)XIC(Port_Data.Port_RW_Complete.[Port])OTU(Port_Data.Port_Write.[Port])OTL(Local_Control.12);
   100: XIC(Local_Control.12)XIO(Port_Data.Port_RW_Complete.[Port])MOV(0,Q90RKU.Command)OTU(Index_Write_Inprocess.[Inprocess_Index])OTU(Local_Control.3)OTU(Command_Being_Processed)OTU(Local_Control.11)OTU(Local_Control.12);
   101: NOP();
   102: EQU(Local_Control,0)XIO(Update_Archive)OTU(Port_Data.Port_Activate.[Port]);
END_ROUTINE
END_ADD_ON_INSTRUCTION
